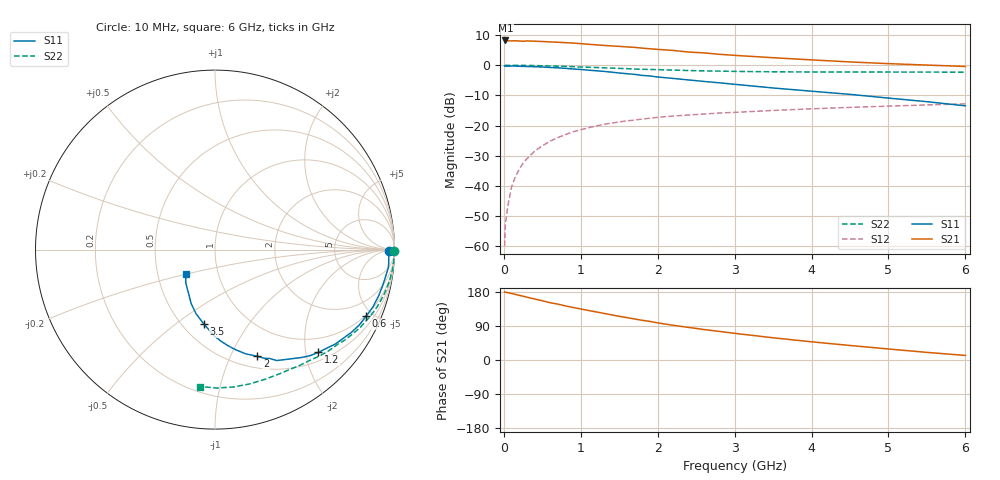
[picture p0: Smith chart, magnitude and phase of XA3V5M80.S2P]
! SIEMENS Discrete & RF Semiconductors
! BFY180
! Si NPN RF Bipolar Junction Transistor in MICRO-X
! VCE = 3.5 V  IC = 0.8 mA
! Common Emitter S-Parameters:  May  1997
# GHz  S  MA  R  50
!  f  S11  S21  S12  S22
! GHz  MAG  ANG  MAG  ANG  MAG  ANG  MAG  ANG
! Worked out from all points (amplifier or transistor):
!   36 points, 10 MHz to 6 GHz, reference 50 ohm
!   highest |S21| = 8.2 dB at 20 MHz (marker M1)
!   |S21| within 3 dB of that: start of sweep to 2.021 GHz
!   unconditionally stable (mu >= 1): 4.387 GHz to end of sweep
!   at 250 MHz: K = 0.07, MSG = 20.2 dB, |S12| = -32.5 dB
!   at 1.4 GHz: K = 0.46, MSG = 12.8 dB, |S12| = -19.2 dB
!   at 6 GHz: K = 1.05, MAG = 4.8 dB, |S12| = -12.8 dB
!   S11 on the Smith chart (normalised r, x): 10 MHz: 59, -13; 600 MHz: 0.94, -4.56; 1.2 GHz: 0.67, -2.26; 2 GHz: 0.63, -1.27; 3.5 GHz: 0.63, -0.64; 6 GHz: 0.70, -0.20
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0.01  0.968 -0.4  2.526 179.5  0.001 89.2  0.9976 -0.3
0.02  0.9679 -0.8  2.581 178.8  0.0023 94.9  0.9999 -0.6
0.05  0.9686 -2.0  2.545 177.8  0.0045 88.2  0.9973 -1.2
0.1  0.971 -4.3  2.537 175.5  0.0096 88.6  0.9977 -2.6
0.2  0.9646 -8.1  2.527 170.6  0.0188 84.2  0.9954 -5.0
0.25  0.9597 -10.1  2.505 168.5  0.0238 82.8  0.9957 -6.4
0.4  0.9474 -15.8  2.511 161.0  0.0375 78.8  0.9887 -9.9
0.6  0.9203 -23.8  2.443 151.3  0.055 72.8  0.9745 -14.8
0.9  0.8685 -34.7  2.337 138.7  0.0788 64.6  0.9481 -21.7
1.1  0.8296 -41.5  2.229 130.7  0.0919 59.8  0.928 -25.8
1.2  0.8122 -44.8  2.185 126.9  0.0987 57.4  0.9189 -28.0
1.5  0.7452 -54.6  2.061 115.2  0.1151 51.2  0.8882 -33.6
1.7  0.7073 -60.9  1.983 108.3  0.1236 47.8  0.8661 -37.1
2  0.6391 -68.4  1.835 97.9  0.1372 43.2  0.8471 -41.9
2.2  0.6055 -73.6  1.763 91.7  0.1439 40.0  0.8323 -45.2
2.6  0.5402 -82.3  1.606 80.4  0.1555 35.3  0.8078 -50.7
3  0.4835 -90.1  1.461 70.4  0.1657 30.8  0.792 -56.1
3.5  0.4203 -98.4  1.335 58.6  0.1781 26.4  0.78 -62.4
4  0.3719 -106.5  1.229 48.0  0.1898 22.1  0.7745 -68.9
4.5  0.3294 -113.8  1.136 38.3  0.2005 17.9  0.7728 -75.5
5.5  0.2491 -130.6  1.008 20.1  0.2201 9.9  0.7712 -89.2
6  0.2124 -140.5  0.956 12.0  0.2292 5.5  0.7675 -96.2
